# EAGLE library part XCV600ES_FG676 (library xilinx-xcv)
xcv600es_fg676 edit this description Auto generated by make-symbol-device-package-bsdl.ulp Rev. 26 Source: xcv600es_fg676.bsd
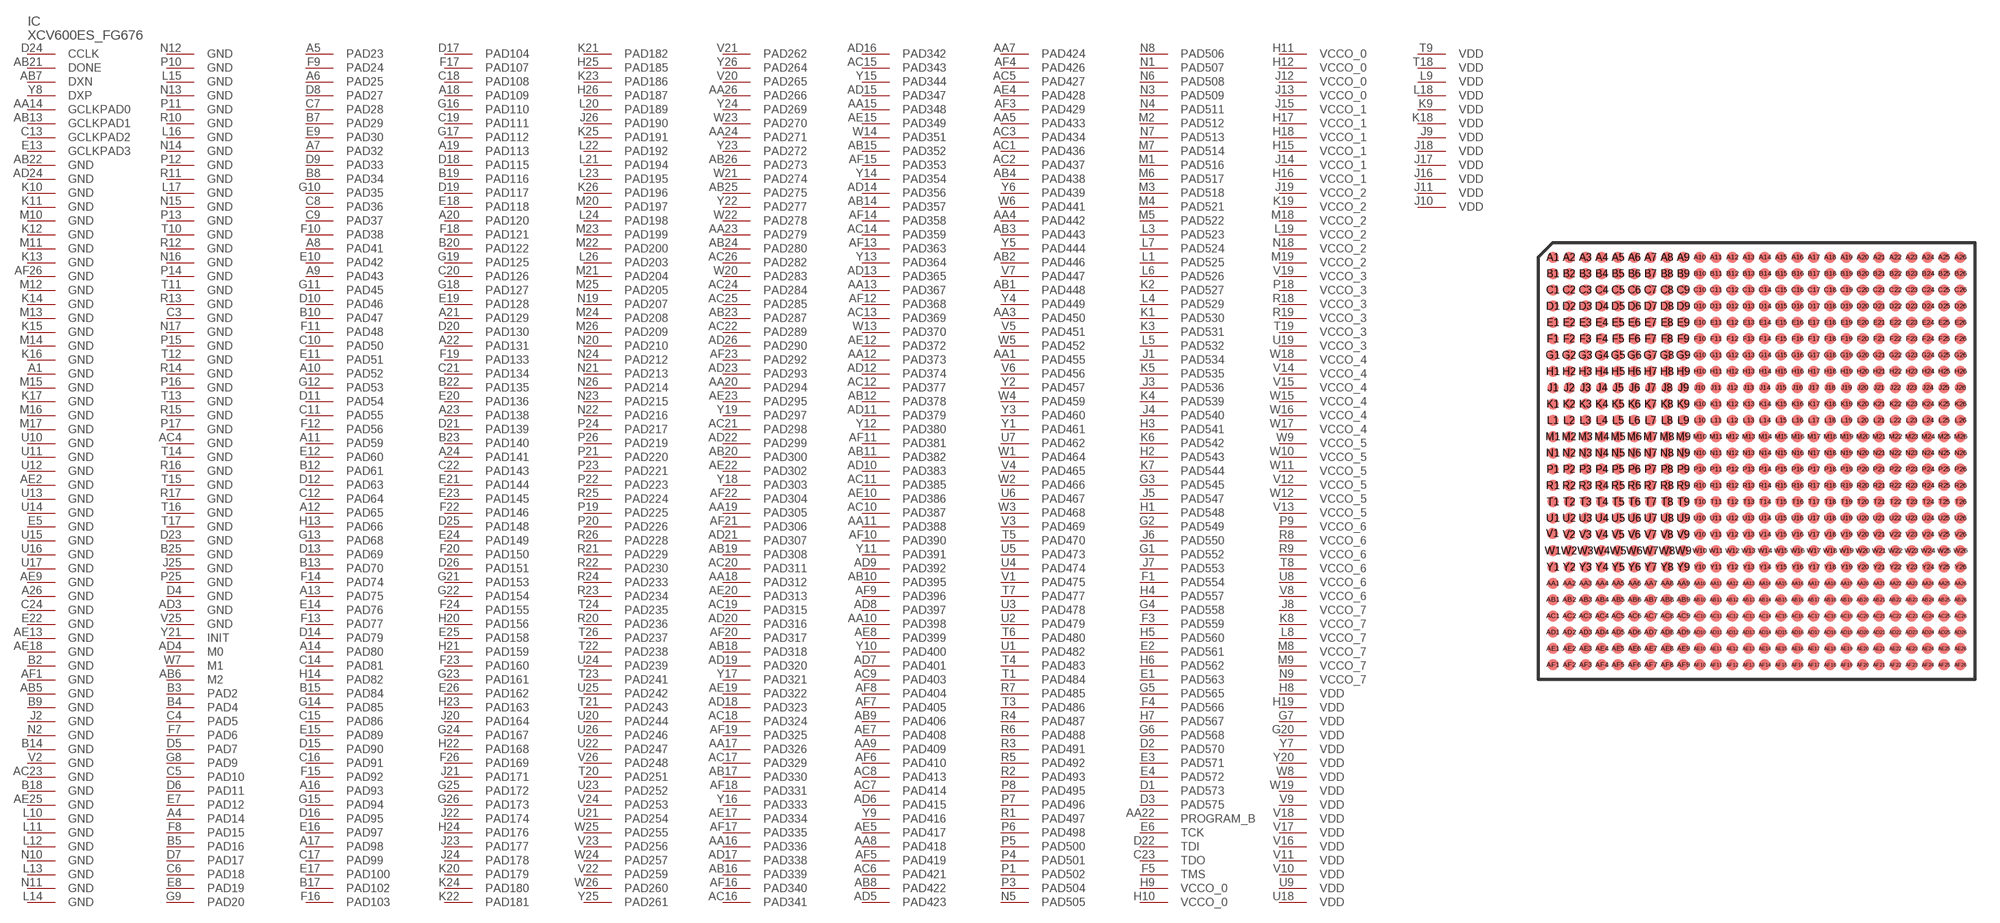
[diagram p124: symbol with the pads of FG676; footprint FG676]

Designator prefix IC

## XCV600ES_FG676 (OC_FARNELL: unknown; OC_NEWARK: unknown)  [FG676]
A1  GND  pwr
A4  PAD14
A5  PAD23
A6  PAD25
A7  PAD32
A8  PAD41
A9  PAD43
A10  PAD52
A11  PAD59
A12  PAD65
A13  PAD75
A14  PAD80
A16  PAD93
A17  PAD98
A18  PAD109
A19  PAD113
A20  PAD120
A21  PAD129
A22  PAD131
A23  PAD138
A24  PAD141
A26  GND  pwr
AA1  PAD455
AA3  PAD450
AA4  PAD442
AA5  PAD433
AA7  PAD424
AA8  PAD418
AA9  PAD409
AA10  PAD398
AA11  PAD388
AA12  PAD373
AA13  PAD367
AA14  GCLKPAD0  in
AA15  PAD348
AA16  PAD336
AA17  PAD326
AA18  PAD312
AA19  PAD305
AA20  PAD294
AA22  PROGRAM_B  in
AA23  PAD279
AA24  PAD271
AA26  PAD266
AB1  PAD448
AB2  PAD446
AB3  PAD443
AB4  PAD438
AB5  GND  pwr
AB6  M2  in
AB7  DXN  pas
AB8  PAD422
AB9  PAD406
AB10  PAD395
AB11  PAD382
AB12  PAD378
AB13  GCLKPAD1  in
AB14  PAD357
AB15  PAD352
AB16  PAD339
AB17  PAD330
AB18  PAD318
AB19  PAD308
AB20  PAD300
AB21  DONE
AB22  GND  pwr
AB23  PAD287
AB24  PAD280
AB25  PAD275
AB26  PAD273
AC1  PAD436
AC2  PAD437
AC3  PAD434
AC4  GND  pwr
AC5  PAD427
AC6  PAD421
AC7  PAD414
AC8  PAD413
AC9  PAD403
AC10  PAD387
AC11  PAD385
AC12  PAD377
AC13  PAD369
AC14  PAD359
AC15  PAD343
AC16  PAD341
AC17  PAD329
AC18  PAD324
AC19  PAD315
AC20  PAD311
AC21  PAD298
AC22  PAD289
AC23  GND  pwr
AC24  PAD284
AC25  PAD285
AC26  PAD282
AD3  GND  pwr
AD4  M0  in
AD5  PAD423
AD6  PAD415
AD7  PAD401
AD8  PAD397
AD9  PAD392
AD10  PAD383
AD11  PAD379
AD12  PAD374
AD13  PAD365
AD14  PAD356
AD15  PAD347
AD16  PAD342
AD17  PAD338
AD18  PAD323
AD19  PAD320
AD20  PAD316
AD21  PAD307
AD22  PAD299
AD23  PAD293
AD24  GND  pwr
AD26  PAD290
AE2  GND  pwr
AE4  PAD428
AE5  PAD417
AE7  PAD408
AE8  PAD399
AE9  GND  pwr
AE10  PAD386
AE12  PAD372
AE13  GND  pwr
AE15  PAD349
AE17  PAD334
AE18  GND  pwr
AE19  PAD322
AE20  PAD313
AE22  PAD302
AE23  PAD295
AE25  GND  pwr
AF1  GND  pwr
AF3  PAD429
AF4  PAD426
AF5  PAD419
AF6  PAD410
AF7  PAD405
AF8  PAD404
AF9  PAD396
AF10  PAD390
AF11  PAD381
AF12  PAD368
AF13  PAD363
AF14  PAD358
AF15  PAD353
AF16  PAD340
AF17  PAD335
AF18  PAD331
AF19  PAD325
AF20  PAD317
AF21  PAD306
AF22  PAD304
AF23  PAD292
AF26  GND  pwr
B2  GND  pwr
B3  PAD2
B4  PAD4
B5  PAD16
B7  PAD29
B8  PAD34
B9  GND  pwr
B10  PAD47
B12  PAD61
B13  PAD70
B14  GND  pwr
B15  PAD84
B17  PAD102
B18  GND  pwr
B19  PAD116
B20  PAD122
B22  PAD135
B23  PAD140
B25  GND  pwr
C3  GND  pwr
C4  PAD5
C5  PAD10
C6  PAD18
C7  PAD28
C8  PAD36
C9  PAD37
C10  PAD50
C11  PAD55
C12  PAD64
C13  GCLKPAD2  in
C14  PAD81
C15  PAD86
C16  PAD91
C17  PAD99
C18  PAD108
C19  PAD111
C20  PAD126
C21  PAD134
C22  PAD143
C23  TDO  out
C24  GND  pwr
D1  PAD573
D2  PAD570
D3  PAD575
D4  GND  pwr
D5  PAD7
D6  PAD11
D7  PAD17
D8  PAD27
D9  PAD33
D10  PAD46
D11  PAD54
D12  PAD63
D13  PAD69
D14  PAD79
D15  PAD90
D16  PAD95
D17  PAD104
D18  PAD115
D19  PAD117
D20  PAD130
D21  PAD139
D22  TDI  in
D23  GND  pwr
D24  CCLK
D25  PAD148
D26  PAD151
E1  PAD563
E2  PAD561
E3  PAD571
E4  PAD572
E5  GND  pwr
E6  TCK  in
E7  PAD12
E8  PAD19
E9  PAD30
E10  PAD42
E11  PAD51
E12  PAD60
E13  GCLKPAD3  in
E14  PAD76
E15  PAD89
E16  PAD97
E17  PAD100
E18  PAD118
E19  PAD128
E20  PAD136
E21  PAD144
E22  GND  pwr
E23  PAD145
E24  PAD149
E25  PAD158
E26  PAD162
F1  PAD554
F3  PAD559
F4  PAD566
F5  TMS  in
F7  PAD6
F8  PAD15
F9  PAD24
F10  PAD38
F11  PAD48
F12  PAD56
F13  PAD77
F14  PAD74
F15  PAD92
F16  PAD103
F17  PAD107
F18  PAD121
F19  PAD133
F20  PAD150
F22  PAD146
F23  PAD160
F24  PAD155
F26  PAD169
G1  PAD552
G2  PAD549
G3  PAD545
G4  PAD558
G5  PAD565
G6  PAD568
G7  VDD  pwr
G8  PAD9
G9  PAD20
G10  PAD35
G11  PAD45
G12  PAD53
G13  PAD68
G14  PAD85
G15  PAD94
G16  PAD110
G17  PAD112
G18  PAD127
G19  PAD125
G20  VDD  pwr
G21  PAD153
G22  PAD154
G23  PAD161
G24  PAD167
G25  PAD172
G26  PAD173
H1  PAD548
H2  PAD543
H3  PAD541
H4  PAD557
H5  PAD560
H6  PAD562
H7  PAD567
H8  VDD  pwr
H9  VCCO_0  pwr
H10  VCCO_0  pwr
H11  VCCO_0  pwr
H12  VCCO_0  pwr
H13  PAD66
H14  PAD82
H15  VCCO_1  pwr
H16  VCCO_1  pwr
H17  VCCO_1  pwr
H18  VCCO_1  pwr
H19  VDD  pwr
H20  PAD156
H21  PAD159
H22  PAD168
H23  PAD163
H24  PAD176
H25  PAD185
H26  PAD187
J1  PAD534
J2  GND  pwr
J3  PAD536
J4  PAD540
J5  PAD547
J6  PAD550
J7  PAD553
J8  VCCO_7  pwr
J9  VDD  pwr
J10  VDD  pwr
J11  VDD  pwr
J12  VCCO_0  pwr
J13  VCCO_0  pwr
J14  VCCO_1  pwr
J15  VCCO_1  pwr
J16  VDD  pwr
J17  VDD  pwr
J18  VDD  pwr
J19  VCCO_2  pwr
J20  PAD164
J21  PAD171
J22  PAD174
J23  PAD177
J24  PAD178
J25  GND  pwr
J26  PAD190
K1  PAD530
K2  PAD527
K3  PAD531
K4  PAD539
K5  PAD535
K6  PAD542
K7  PAD544
K8  VCCO_7  pwr
K9  VDD  pwr
K10  GND  pwr
K11  GND  pwr
K12  GND  pwr
K13  GND  pwr
K14  GND  pwr
K15  GND  pwr
K16  GND  pwr
K17  GND  pwr
K18  VDD  pwr
K19  VCCO_2  pwr
K20  PAD179
K21  PAD182
K22  PAD181
K23  PAD186
K24  PAD180
K25  PAD191
K26  PAD196
L1  PAD525
L3  PAD523
L4  PAD529
L5  PAD532
L6  PAD526
L7  PAD524
L8  VCCO_7  pwr
L9  VDD  pwr
L10  GND  pwr
L11  GND  pwr
L12  GND  pwr
L13  GND  pwr
L14  GND  pwr
L15  GND  pwr
L16  GND  pwr
L17  GND  pwr
L18  VDD  pwr
L19  VCCO_2  pwr
L20  PAD189
L21  PAD194
L22  PAD192
L23  PAD195
L24  PAD198
L26  PAD203
M1  PAD516
M2  PAD512
M3  PAD518
M4  PAD521
M5  PAD522
M6  PAD517
M7  PAD514
M8  VCCO_7  pwr
M9  VCCO_7  pwr
M10  GND  pwr
M11  GND  pwr
M12  GND  pwr
M13  GND  pwr
M14  GND  pwr
M15  GND  pwr
M16  GND  pwr
M17  GND  pwr
M18  VCCO_2  pwr
M19  VCCO_2  pwr
M20  PAD197
M21  PAD204
M22  PAD200
M23  PAD199
M24  PAD208
M25  PAD205
M26  PAD209
N1  PAD507
N2  GND  pwr
N3  PAD509
N4  PAD511
N5  PAD505
N6  PAD508
N7  PAD513
N8  PAD506
N9  VCCO_7  pwr
N10  GND  pwr
N11  GND  pwr
N12  GND  pwr
N13  GND  pwr
N14  GND  pwr
N15  GND  pwr
N16  GND  pwr
N17  GND  pwr
N18  VCCO_2  pwr
N19  PAD207
N20  PAD210
N21  PAD213
N22  PAD216
N23  PAD215
N24  PAD212
N26  PAD214
P1  PAD502
P3  PAD504
P4  PAD501
P5  PAD500
P6  PAD498
P7  PAD496
P8  PAD495
P9  VCCO_6  pwr
P10  GND  pwr
P11  GND  pwr
P12  GND  pwr
P13  GND  pwr
P14  GND  pwr
P15  GND  pwr
P16  GND  pwr
P17  GND  pwr
P18  VCCO_3  pwr
P19  PAD225
P20  PAD226
P21  PAD220
P22  PAD223
P23  PAD221
P24  PAD217
P25  GND  pwr
P26  PAD219
R1  PAD497
R2  PAD493
R3  PAD491
R4  PAD487
R5  PAD492
R6  PAD488
R7  PAD485
R8  VCCO_6  pwr
R9  VCCO_6  pwr
R10  GND  pwr
R11  GND  pwr
R12  GND  pwr
R13  GND  pwr
R14  GND  pwr
R15  GND  pwr
R16  GND  pwr
R17  GND  pwr
R18  VCCO_3  pwr
R19  VCCO_3  pwr
R20  PAD236
R21  PAD229
R22  PAD230
R23  PAD234
R24  PAD233
R25  PAD224
R26  PAD228
T1  PAD484
T3  PAD486
T4  PAD483
T5  PAD470
T6  PAD480
T7  PAD477
T8  VCCO_6  pwr
T9  VDD  pwr
T10  GND  pwr
T11  GND  pwr
T12  GND  pwr
T13  GND  pwr
T14  GND  pwr
T15  GND  pwr
T16  GND  pwr
T17  GND  pwr
T18  VDD  pwr
T19  VCCO_3  pwr
T20  PAD251
T21  PAD243
T22  PAD238
T23  PAD241
T24  PAD235
T26  PAD237
U1  PAD482
U2  PAD479
U3  PAD478
U4  PAD474
U5  PAD473
U6  PAD467
U7  PAD462
U8  VCCO_6  pwr
U9  VDD  pwr
U10  GND  pwr
U11  GND  pwr
U12  GND  pwr
U13  GND  pwr
U14  GND  pwr
U15  GND  pwr
U16  GND  pwr
U17  GND  pwr
U18  VDD  pwr
U19  VCCO_3  pwr
U20  PAD244
U21  PAD254
U22  PAD247
U23  PAD252
U24  PAD239
U25  PAD242
U26  PAD246
V1  PAD475
V2  GND  pwr
V3  PAD469
V4  PAD465
V5  PAD451
V6  PAD456
V7  PAD447
V8  VCCO_6  pwr
V9  VDD  pwr
V10  VDD  pwr
V11  VDD  pwr
V12  VCCO_5  pwr
V13  VCCO_5  pwr
V14  VCCO_4  pwr
V15  VCCO_4  pwr
V16  VDD  pwr
V17  VDD  pwr
V18  VDD  pwr
V19  VCCO_3  pwr
V20  PAD265
V21  PAD262
V22  PAD259
V23  PAD256
V24  PAD253
V25  GND  pwr
V26  PAD248
W1  PAD464
W2  PAD466
W3  PAD468
W4  PAD459
W5  PAD452
W6  PAD441
W7  M1  in
W8  VDD  pwr
W9  VCCO_5  pwr
W10  VCCO_5  pwr
W11  VCCO_5  pwr
W12  VCCO_5  pwr
W13  PAD370
W14  PAD351
W15  VCCO_4  pwr
W16  VCCO_4  pwr
W17  VCCO_4  pwr
W18  VCCO_4  pwr
W19  VDD  pwr
W20  PAD283
W21  PAD274
W22  PAD278
W23  PAD270
W24  PAD257
W25  PAD255
W26  PAD260
Y1  PAD461
Y2  PAD457
Y3  PAD460
Y4  PAD449
Y5  PAD444
Y6  PAD439
Y7  VDD  pwr
Y8  DXP  pas
Y9  PAD416
Y10  PAD400
Y11  PAD391
Y12  PAD380
Y13  PAD364
Y14  PAD354
Y15  PAD344
Y16  PAD333
Y17  PAD321
Y18  PAD303
Y19  PAD297
Y20  VDD  pwr
Y21  INIT
Y22  PAD277
Y23  PAD272
Y24  PAD269
Y25  PAD261
Y26  PAD264

## Footprint FG676 (pad centres in mm)
xcv400_fg676 edit this description Auto generated by make-symbol-device-package-bsdl.ulp Rev. 26 Source: xcv400_fg676.bsd
smd 0.7 x 0.7: A1 -12.5,12.5; A2 -11.5,12.5; A3 -10.5,12.5; A4 -9.5,12.5; A5 -8.5,12.5; A6 -7.5,12.5; A7 -6.5,12.5; A8 -5.5,12.5; A9 -4.5,12.5; A10 -3.5,12.5; A11 -2.5,12.5; A12 -1.5,12.5; A13 -0.5,12.5; A14 0.5,12.5; A15 1.5,12.5; A16 2.5,12.5; A17 3.5,12.5; A18 4.5,12.5; A19 5.5,12.5; A20 6.5,12.5; A21 7.5,12.5; A22 8.5,12.5; A23 9.5,12.5; A24 10.5,12.5; A25 11.5,12.5; A26 12.5,12.5; AA1 -12.5,-7.5; AA2 -11.5,-7.5; AA3 -10.5,-7.5; AA4 -9.5,-7.5; AA5 -8.5,-7.5; AA6 -7.5,-7.5; AA7 -6.5,-7.5; AA8 -5.5,-7.5; AA9 -4.5,-7.5; AA10 -3.5,-7.5; AA11 -2.5,-7.5; AA12 -1.5,-7.5; AA13 -0.5,-7.5; AA14 0.5,-7.5; AA15 1.5,-7.5; AA16 2.5,-7.5; AA17 3.5,-7.5; AA18 4.5,-7.5; AA19 5.5,-7.5; AA20 6.5,-7.5; AA21 7.5,-7.5; AA22 8.5,-7.5; AA23 9.5,-7.5; AA24 10.5,-7.5; AA25 11.5,-7.5; AA26 12.5,-7.5; AB1 -12.5,-8.5; AB2 -11.5,-8.5; AB3 -10.5,-8.5; AB4 -9.5,-8.5; AB5 -8.5,-8.5; AB6 -7.5,-8.5; AB7 -6.5,-8.5; AB8 -5.5,-8.5; AB9 -4.5,-8.5; AB10 -3.5,-8.5; AB11 -2.5,-8.5; AB12 -1.5,-8.5; AB13 -0.5,-8.5; AB14 0.5,-8.5; AB15 1.5,-8.5; AB16 2.5,-8.5; AB17 3.5,-8.5; AB18 4.5,-8.5; AB19 5.5,-8.5; AB20 6.5,-8.5; AB21 7.5,-8.5; AB22 8.5,-8.5; AB23 9.5,-8.5; AB24 10.5,-8.5; AB25 11.5,-8.5; AB26 12.5,-8.5; AC1 -12.5,-9.5; AC2 -11.5,-9.5; AC3 -10.5,-9.5; AC4 -9.5,-9.5; AC5 -8.5,-9.5; AC6 -7.5,-9.5; AC7 -6.5,-9.5; AC8 -5.5,-9.5; AC9 -4.5,-9.5; AC10 -3.5,-9.5; AC11 -2.5,-9.5; AC12 -1.5,-9.5; AC13 -0.5,-9.5; AC14 0.5,-9.5; AC15 1.5,-9.5; AC16 2.5,-9.5; AC17 3.5,-9.5; AC18 4.5,-9.5; AC19 5.5,-9.5; AC20 6.5,-9.5; AC21 7.5,-9.5; AC22 8.5,-9.5; AC23 9.5,-9.5; AC24 10.5,-9.5; AC25 11.5,-9.5; AC26 12.5,-9.5; AD1 -12.5,-10.5; AD2 -11.5,-10.5; AD3 -10.5,-10.5; AD4 -9.5,-10.5; AD5 -8.5,-10.5; AD6 -7.5,-10.5; AD7 -6.5,-10.5; AD8 -5.5,-10.5; AD9 -4.5,-10.5; AD10 -3.5,-10.5; AD11 -2.5,-10.5; AD12 -1.5,-10.5; AD13 -0.5,-10.5; AD14 0.5,-10.5; AD15 1.5,-10.5; AD16 2.5,-10.5; AD17 3.5,-10.5; AD18 4.5,-10.5; AD19 5.5,-10.5; AD20 6.5,-10.5; AD21 7.5,-10.5; AD22 8.5,-10.5; AD23 9.5,-10.5; AD24 10.5,-10.5; AD25 11.5,-10.5; AD26 12.5,-10.5; AE1 -12.5,-11.5; AE2 -11.5,-11.5; AE3 -10.5,-11.5; AE4 -9.5,-11.5; AE5 -8.5,-11.5; AE6 -7.5,-11.5; AE7 -6.5,-11.5; AE8 -5.5,-11.5; AE9 -4.5,-11.5; AE10 -3.5,-11.5; AE11 -2.5,-11.5; AE12 -1.5,-11.5; AE13 -0.5,-11.5; AE14 0.5,-11.5; AE15 1.5,-11.5; AE16 2.5,-11.5; AE17 3.5,-11.5; AE18 4.5,-11.5; AE19 5.5,-11.5; AE20 6.5,-11.5; AE21 7.5,-11.5; AE22 8.5,-11.5; AE23 9.5,-11.5; AE24 10.5,-11.5; AE25 11.5,-11.5; AE26 12.5,-11.5; AF1 -12.5,-12.5; AF2 -11.5,-12.5; AF3 -10.5,-12.5; AF4 -9.5,-12.5; AF5 -8.5,-12.5; AF6 -7.5,-12.5; AF7 -6.5,-12.5; AF8 -5.5,-12.5; AF9 -4.5,-12.5; AF10 -3.5,-12.5; AF11 -2.5,-12.5; AF12 -1.5,-12.5; AF13 -0.5,-12.5; AF14 0.5,-12.5; AF15 1.5,-12.5; AF16 2.5,-12.5; AF17 3.5,-12.5; AF18 4.5,-12.5; AF19 5.5,-12.5; AF20 6.5,-12.5; AF21 7.5,-12.5; AF22 8.5,-12.5; AF23 9.5,-12.5; AF24 10.5,-12.5; AF25 11.5,-12.5; AF26 12.5,-12.5; B1 -12.5,11.5; B2 -11.5,11.5; B3 -10.5,11.5; B4 -9.5,11.5; B5 -8.5,11.5; B6 -7.5,11.5; B7 -6.5,11.5; B8 -5.5,11.5; B9 -4.5,11.5; B10 -3.5,11.5; B11 -2.5,11.5; B12 -1.5,11.5; B13 -0.5,11.5; B14 0.5,11.5; B15 1.5,11.5; B16 2.5,11.5; B17 3.5,11.5; B18 4.5,11.5; B19 5.5,11.5; B20 6.5,11.5; B21 7.5,11.5; B22 8.5,11.5; B23 9.5,11.5; B24 10.5,11.5; B25 11.5,11.5; B26 12.5,11.5; C1 -12.5,10.5; C2 -11.5,10.5; C3 -10.5,10.5; C4 -9.5,10.5; C5 -8.5,10.5; C6 -7.5,10.5; C7 -6.5,10.5; C8 -5.5,10.5; C9 -4.5,10.5; C10 -3.5,10.5; C11 -2.5,10.5; C12 -1.5,10.5; C13 -0.5,10.5; C14 0.5,10.5; C15 1.5,10.5; C16 2.5,10.5; C17 3.5,10.5; C18 4.5,10.5; C19 5.5,10.5; C20 6.5,10.5; C21 7.5,10.5; C22 8.5,10.5; C23 9.5,10.5; C24 10.5,10.5; C25 11.5,10.5; C26 12.5,10.5; D1 -12.5,9.5; D2 -11.5,9.5; D3 -10.5,9.5; D4 -9.5,9.5; D5 -8.5,9.5; D6 -7.5,9.5; D7 -6.5,9.5; D8 -5.5,9.5; D9 -4.5,9.5; D10 -3.5,9.5; D11 -2.5,9.5; D12 -1.5,9.5; D13 -0.5,9.5; D14 0.5,9.5; D15 1.5,9.5; D16 2.5,9.5; D17 3.5,9.5; D18 4.5,9.5; D19 5.5,9.5; D20 6.5,9.5; D21 7.5,9.5; D22 8.5,9.5; D23 9.5,9.5; D24 10.5,9.5; D25 11.5,9.5; D26 12.5,9.5; E1 -12.5,8.5; E2 -11.5,8.5; E3 -10.5,8.5; E4 -9.5,8.5; E5 -8.5,8.5; E6 -7.5,8.5; E7 -6.5,8.5; E8 -5.5,8.5; E9 -4.5,8.5; E10 -3.5,8.5; E11 -2.5,8.5; E12 -1.5,8.5; E13 -0.5,8.5; E14 0.5,8.5; E15 1.5,8.5; E16 2.5,8.5; E17 3.5,8.5; E18 4.5,8.5; E19 5.5,8.5; E20 6.5,8.5; E21 7.5,8.5; E22 8.5,8.5; E23 9.5,8.5; E24 10.5,8.5; E25 11.5,8.5; E26 12.5,8.5; F1 -12.5,7.5; F2 -11.5,7.5; F3 -10.5,7.5; F4 -9.5,7.5; F5 -8.5,7.5; F6 -7.5,7.5; F7 -6.5,7.5; F8 -5.5,7.5; F9 -4.5,7.5; F10 -3.5,7.5; F11 -2.5,7.5; F12 -1.5,7.5; F13 -0.5,7.5; F14 0.5,7.5; F15 1.5,7.5; F16 2.5,7.5; F17 3.5,7.5; F18 4.5,7.5; F19 5.5,7.5; F20 6.5,7.5; F21 7.5,7.5; F22 8.5,7.5; F23 9.5,7.5; F24 10.5,7.5; F25 11.5,7.5; F26 12.5,7.5; G1 -12.5,6.5; G2 -11.5,6.5; G3 -10.5,6.5; G4 -9.5,6.5; G5 -8.5,6.5; G6 -7.5,6.5; G7 -6.5,6.5; G8 -5.5,6.5; G9 -4.5,6.5; G10 -3.5,6.5; G11 -2.5,6.5; G12 -1.5,6.5; G13 -0.5,6.5; G14 0.5,6.5; G15 1.5,6.5; G16 2.5,6.5; G17 3.5,6.5; G18 4.5,6.5; G19 5.5,6.5; G20 6.5,6.5; G21 7.5,6.5; G22 8.5,6.5; G23 9.5,6.5; G24 10.5,6.5; G25 11.5,6.5; G26 12.5,6.5; H1 -12.5,5.5; H2 -11.5,5.5; H3 -10.5,5.5; H4 -9.5,5.5; H5 -8.5,5.5; H6 -7.5,5.5; H7 -6.5,5.5; H8 -5.5,5.5; H9 -4.5,5.5; H10 -3.5,5.5; H11 -2.5,5.5; H12 -1.5,5.5; H13 -0.5,5.5; H14 0.5,5.5; H15 1.5,5.5; H16 2.5,5.5; H17 3.5,5.5; H18 4.5,5.5; H19 5.5,5.5; H20 6.5,5.5; H21 7.5,5.5; H22 8.5,5.5; H23 9.5,5.5; H24 10.5,5.5; H25 11.5,5.5; H26 12.5,5.5; J1 -12.5,4.5; J2 -11.5,4.5; J3 -10.5,4.5; J4 -9.5,4.5; J5 -8.5,4.5; J6 -7.5,4.5; J7 -6.5,4.5; J8 -5.5,4.5; J9 -4.5,4.5; J10 -3.5,4.5; J11 -2.5,4.5; J12 -1.5,4.5; J13 -0.5,4.5; J14 0.5,4.5; J15 1.5,4.5; J16 2.5,4.5; J17 3.5,4.5; J18 4.5,4.5; J19 5.5,4.5; J20 6.5,4.5; J21 7.5,4.5; J22 8.5,4.5; J23 9.5,4.5; J24 10.5,4.5; J25 11.5,4.5; J26 12.5,4.5; K1 -12.5,3.5; K2 -11.5,3.5; K3 -10.5,3.5; K4 -9.5,3.5; K5 -8.5,3.5; K6 -7.5,3.5; K7 -6.5,3.5; K8 -5.5,3.5; K9 -4.5,3.5; K10 -3.5,3.5; K11 -2.5,3.5; K12 -1.5,3.5; K13 -0.5,3.5; K14 0.5,3.5; K15 1.5,3.5; K16 2.5,3.5; K17 3.5,3.5; K18 4.5,3.5; K19 5.5,3.5; K20 6.5,3.5; K21 7.5,3.5; K22 8.5,3.5; K23 9.5,3.5; K24 10.5,3.5; K25 11.5,3.5; K26 12.5,3.5; L1 -12.5,2.5; L2 -11.5,2.5; L3 -10.5,2.5; L4 -9.5,2.5; L5 -8.5,2.5; L6 -7.5,2.5; L7 -6.5,2.5; L8 -5.5,2.5; L9 -4.5,2.5; L10 -3.5,2.5; L11 -2.5,2.5; L12 -1.5,2.5; L13 -0.5,2.5; L14 0.5,2.5; L15 1.5,2.5; L16 2.5,2.5; L17 3.5,2.5; L18 4.5,2.5; L19 5.5,2.5; L20 6.5,2.5; L21 7.5,2.5; L22 8.5,2.5; L23 9.5,2.5; L24 10.5,2.5; L25 11.5,2.5; L26 12.5,2.5; M1 -12.5,1.5; M2 -11.5,1.5; M3 -10.5,1.5; M4 -9.5,1.5; M5 -8.5,1.5; M6 -7.5,1.5; M7 -6.5,1.5; M8 -5.5,1.5; M9 -4.5,1.5; M10 -3.5,1.5; M11 -2.5,1.5; M12 -1.5,1.5; M13 -0.5,1.5; M14 0.5,1.5; M15 1.5,1.5; M16 2.5,1.5; M17 3.5,1.5; M18 4.5,1.5; M19 5.5,1.5; M20 6.5,1.5; M21 7.5,1.5; M22 8.5,1.5; M23 9.5,1.5; M24 10.5,1.5; M25 11.5,1.5; M26 12.5,1.5; N1 -12.5,0.5; N2 -11.5,0.5; N3 -10.5,0.5; N4 -9.5,0.5; N5 -8.5,0.5; N6 -7.5,0.5; N7 -6.5,0.5; N8 -5.5,0.5; N9 -4.5,0.5; N10 -3.5,0.5; N11 -2.5,0.5; N12 -1.5,0.5; N13 -0.5,0.5; N14 0.5,0.5; N15 1.5,0.5; N16 2.5,0.5; N17 3.5,0.5; N18 4.5,0.5; N19 5.5,0.5; N20 6.5,0.5; N21 7.5,0.5; N22 8.5,0.5; N23 9.5,0.5; N24 10.5,0.5; N25 11.5,0.5; N26 12.5,0.5; P1 -12.5,-0.5; P2 -11.5,-0.5; P3 -10.5,-0.5; P4 -9.5,-0.5; P5 -8.5,-0.5; P6 -7.5,-0.5; P7 -6.5,-0.5; P8 -5.5,-0.5; P9 -4.5,-0.5; P10 -3.5,-0.5; P11 -2.5,-0.5; P12 -1.5,-0.5; P13 -0.5,-0.5; P14 0.5,-0.5; P15 1.5,-0.5; P16 2.5,-0.5; P17 3.5,-0.5; P18 4.5,-0.5; P19 5.5,-0.5; P20 6.5,-0.5; P21 7.5,-0.5; P22 8.5,-0.5; P23 9.5,-0.5; P24 10.5,-0.5; P25 11.5,-0.5; P26 12.5,-0.5; R1 -12.5,-1.5; R2 -11.5,-1.5; R3 -10.5,-1.5; R4 -9.5,-1.5; R5 -8.5,-1.5; R6 -7.5,-1.5; R7 -6.5,-1.5; R8 -5.5,-1.5; R9 -4.5,-1.5; R10 -3.5,-1.5; R11 -2.5,-1.5; R12 -1.5,-1.5; R13 -0.5,-1.5; R14 0.5,-1.5; R15 1.5,-1.5; R16 2.5,-1.5; R17 3.5,-1.5; R18 4.5,-1.5; R19 5.5,-1.5; R20 6.5,-1.5; R21 7.5,-1.5; R22 8.5,-1.5; R23 9.5,-1.5; R24 10.5,-1.5; R25 11.5,-1.5; R26 12.5,-1.5; T1 -12.5,-2.5; T2 -11.5,-2.5; T3 -10.5,-2.5; T4 -9.5,-2.5; T5 -8.5,-2.5; T6 -7.5,-2.5; T7 -6.5,-2.5; T8 -5.5,-2.5; T9 -4.5,-2.5; T10 -3.5,-2.5; T11 -2.5,-2.5; T12 -1.5,-2.5; T13 -0.5,-2.5; T14 0.5,-2.5; T15 1.5,-2.5; T16 2.5,-2.5; T17 3.5,-2.5; T18 4.5,-2.5; T19 5.5,-2.5; T20 6.5,-2.5; T21 7.5,-2.5; T22 8.5,-2.5; T23 9.5,-2.5; T24 10.5,-2.5; T25 11.5,-2.5; T26 12.5,-2.5; U1 -12.5,-3.5; U2 -11.5,-3.5; U3 -10.5,-3.5; U4 -9.5,-3.5; U5 -8.5,-3.5; U6 -7.5,-3.5; U7 -6.5,-3.5; U8 -5.5,-3.5; U9 -4.5,-3.5; U10 -3.5,-3.5; U11 -2.5,-3.5; U12 -1.5,-3.5; U13 -0.5,-3.5; U14 0.5,-3.5; U15 1.5,-3.5; U16 2.5,-3.5; U17 3.5,-3.5; U18 4.5,-3.5; U19 5.5,-3.5; U20 6.5,-3.5; U21 7.5,-3.5; U22 8.5,-3.5; U23 9.5,-3.5; U24 10.5,-3.5; U25 11.5,-3.5; U26 12.5,-3.5; V1 -12.527,-4.431; V2 -11.5,-4.5; V3 -10.5,-4.5; V4 -9.5,-4.5; V5 -8.5,-4.5; V6 -7.5,-4.5; V7 -6.5,-4.5; V8 -5.5,-4.5; V9 -4.5,-4.5; V10 -3.5,-4.5; V11 -2.5,-4.5; V12 -1.5,-4.5; V13 -0.5,-4.5; V14 0.5,-4.5; V15 1.5,-4.5; V16 2.5,-4.5; V17 3.5,-4.5; V18 4.5,-4.5; V19 5.5,-4.5; V20 6.5,-4.5; V21 7.5,-4.5; V22 8.5,-4.5; V23 9.5,-4.5; V24 10.5,-4.5; V25 11.5,-4.5; V26 12.5,-4.5; W1 -12.5,-5.5; W2 -11.5,-5.5; W3 -10.5,-5.5; W4 -9.5,-5.5; W5 -8.5,-5.5; W6 -7.5,-5.5; W7 -6.5,-5.5; W8 -5.5,-5.5; W9 -4.5,-5.5; W10 -3.5,-5.5; W11 -2.5,-5.5; W12 -1.5,-5.5; W13 -0.5,-5.5; W14 0.5,-5.5; W15 1.5,-5.5; W16 2.5,-5.5; W17 3.5,-5.5; W18 4.5,-5.5; W19 5.5,-5.5; W20 6.5,-5.5; W21 7.5,-5.5; W22 8.5,-5.5; W23 9.5,-5.5; W24 10.5,-5.5; W25 11.5,-5.5; W26 12.5,-5.5; Y1 -12.5,-6.5; Y2 -11.5,-6.5; Y3 -10.5,-6.5; Y4 -9.5,-6.5; Y5 -8.5,-6.5; Y6 -7.5,-6.5; Y7 -6.5,-6.5; Y8 -5.5,-6.5; Y9 -4.5,-6.5; Y10 -3.5,-6.5; Y11 -2.5,-6.5; Y12 -1.5,-6.5; Y13 -0.5,-6.5; Y14 0.5,-6.5; Y15 1.5,-6.5; Y16 2.5,-6.5; Y17 3.5,-6.5; Y18 4.5,-6.5; Y19 5.5,-6.5; Y20 6.5,-6.5; Y21 7.5,-6.5; Y22 8.5,-6.5; Y23 9.5,-6.5; Y24 10.5,-6.5; Y25 11.5,-6.5; Y26 12.5,-6.5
